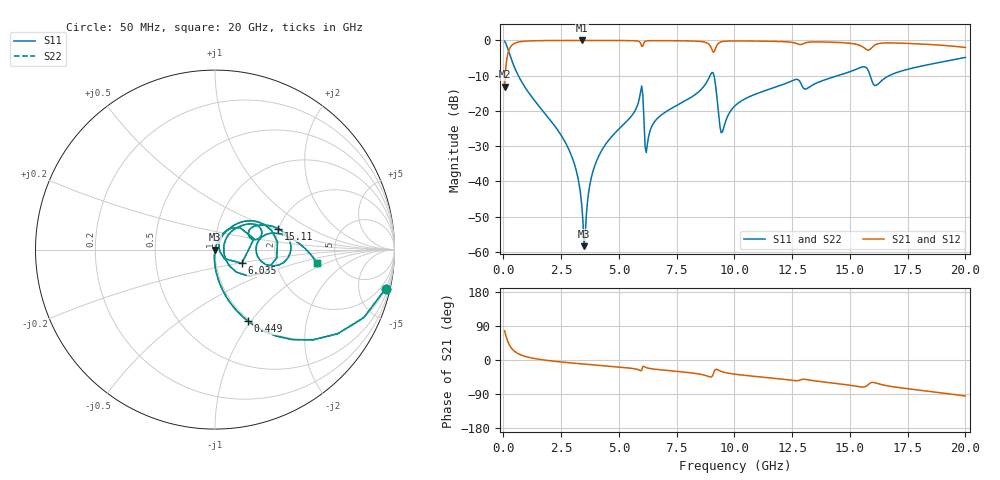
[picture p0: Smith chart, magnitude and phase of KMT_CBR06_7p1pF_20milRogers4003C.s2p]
! Data measured by Modelithics Inc. support@modelithics.com 813-866-6335
! KEMET CBR0603 7.1pF, Pad Width= 0.851mm, Pad Length= 0.64mm, Pad Gap= 0.62mm, 20mil Rogers 4003C substrate Data, January 2022
# hz S ma R 50
! 2 Port Network Data from SP1.SP block
! freq  magS11  angS11  magS21  angS21  magS12  angS12  magS22  angS22
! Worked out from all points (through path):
!   401 points, 50 MHz to 20 GHz, reference 50 ohm
!   highest |S21| = -0.01 dB at 3.392 GHz (marker M1); lowest = -13.2 dB at 50 MHz (marker M2)
!   group delay of S21, straight-line fit = 14.2 ps
!   lowest |S11| = -58.4 dB at 3.491 GHz (marker M3), VSWR 1.00, Z = 50.1 - j0.0743 ohm
!   |S11| at or under -10 dB: 644.8 MHz to 8.945 GHz (8.3 GHz wide, 173 % of centre); 9.116 GHz to 14.48 GHz (5.368 GHz wide, 45.5 % of centre); 15.88 GHz to 16.7 GHz (821.9 MHz wide, 5.05 % of centre)
!   |S22| runs from -58.4 to -0.2 dB; largest |S21 - S12| = 0
!   S11 on the Smith chart (normalised r, x): 50 MHz: 0.98, -8.78; 449 MHz: 0.98, -0.96; 6.035 GHz: 1.33, -0.21; 15.11 GHz: 1.99, +0.54; 20 GHz: 3.50, -0.79
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5e7  0.9755 -12.8  0.2196 77.1  0.2196 77.1  0.9755 -12.8
2.495e8  0.6629 -49.2  0.7481 40.7  0.7481 40.7  0.6629 -49.2
4.49e8  0.4377 -65.4  0.8985 24.6  0.8985 24.6  0.4377 -65.4
2.793125e9  0.03019 -95.1  0.9985 -6.9  0.9985 -6.9  0.03019 -95.1
3.192125e9  0.01257 -94.5  0.9988 -9.2  0.9988 -9.2  0.01257 -94.5
3.391625e9  0.004574 -86.9  0.9988 -10.3  0.9988 -10.3  0.004574 -86.9
3.491375e9  0.001206 -37.9  0.9988 -10.8  0.9988 -10.8  0.001206 -37.9
3.790625e9  0.0108 71.6  0.9987 -12.4  0.9987 -12.4  0.0108 71.6
4.13975e9  0.02343 72.9  0.9984 -14.2  0.9984 -14.2  0.02343 72.9
5.93525e9  0.1848 41.7  0.9216 -28.3  0.9216 -28.3  0.1848 41.7
6.035e9  0.168 -26.9  0.8339 -17.0  0.8339 -17.0  0.168 -26.9
6.2345e9  0.03453 48.8  0.9874 -21.1  0.9874 -21.1  0.03453 48.8
6.73325e9  0.08223 62.4  0.9934 -25.5  0.9934 -25.5  0.08223 62.4
9.0275e9  0.3508 7.3  0.7406 -43.5  0.7406 -43.5  0.3508 7.3
9.4265e9  0.04908 -7.8  0.9541 -30.0  0.9541 -30.0  0.04908 -7.8
1.0025e10  0.1182 47.9  0.9833 -37.5  0.9833 -37.5  0.1182 47.9
1.26185e10  0.2775 27.2  0.9209 -54.4  0.9209 -54.4  0.2775 27.2
1.336662e10  0.2313 30.7  0.9516 -54.0  0.9516 -54.0  0.2313 30.7
1.511225e10  0.3711 18.4  0.9023 -67.6  0.9023 -67.6  0.3711 18.4
1.586038e10  0.3295 -16.2  0.7404 -61.7  0.7404 -61.7  0.3295 -16.2
1.670825e10  0.3172 16.4  0.9229 -69.0  0.9229 -69.0  0.3172 16.4
2e10  0.5739 -7.6  0.7936 -95.1  0.7936 -95.1  0.5739 -7.6
